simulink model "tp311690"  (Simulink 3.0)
settings: Solver=ode45  StartTime=0.0  StopTime=1  RelTol=1e-3

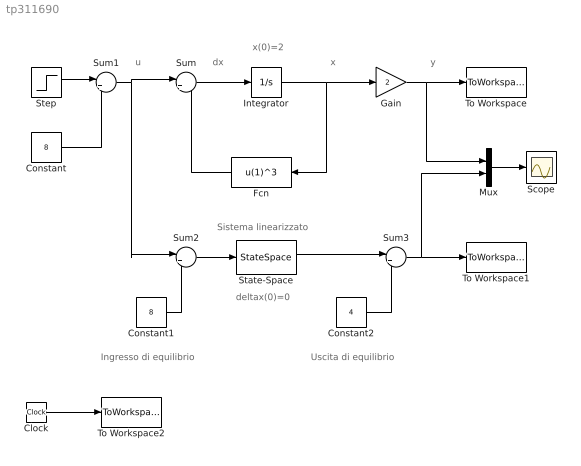
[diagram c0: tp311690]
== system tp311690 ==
  note: dx
  note: x
  note: y
  note: Sistema linearizzato
  note: x(0)=2
  note: deltax(0)=0
  note: Ingresso di equilibrio
  note: Uscita di equilibrio
  note: u
  Clock : Clock
  Constant : Constant  Value=8
  Constant1 : Constant  Value=8
  Constant2 : Constant  Value=4
  Fcn : Fcn  Orientation=left  Expr=u(1)^3
  Gain : Gain  Gain=2  SaturateOnIntegerOverflow=on
  Integrator : Integrator  ExternalReset=none  InitialConditionSource=internal  InitialCondition=2  LimitOutput=off  UpperSaturationLimit=inf  LowerSaturationLimit=-inf  ShowSaturationPort=off  ShowStatePort=off  AbsoluteTolerance=auto
  Mux : Mux  Inputs=2
  Scope : Scope
  State-Space : StateSpace  A=-12  B=1  C=2  D=0  X0=0
  Step : Step  Time=0.1  Before=0  After=1  SampleTime=0
  Sum : Sum  Inputs=|+-  SaturateOnIntegerOverflow=on
  Sum1 : Sum  Inputs=|++  SaturateOnIntegerOverflow=on
  Sum2 : Sum  Inputs=|+-  SaturateOnIntegerOverflow=on
  Sum3 : Sum  Inputs=|++  SaturateOnIntegerOverflow=on
  To Workspace : ToWorkspace  VariableName=y  SampleTime=-1  SaveFormat=Matrix
  To Workspace1 : ToWorkspace  VariableName=yl  SampleTime=-1  SaveFormat=Matrix
  To Workspace2 : ToWorkspace  VariableName=t  SampleTime=-1  SaveFormat=Matrix
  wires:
  Integrator/1 -> Gain/1, Fcn/1
  Sum/1 -> Integrator/1
  Gain/1 -> To Workspace/1, Mux/1
  Fcn/1 -> Sum/2
  Clock/1 -> To Workspace2/1
  Step/1 -> Sum1/1
  Sum1/1 -> Sum/1, Sum2/1
  Constant/1 -> Sum1/2
  Constant1/1 -> Sum2/2
  Sum2/1 -> State-Space/1
  State-Space/1 -> Sum3/1
  Constant2/1 -> Sum3/2
  Sum3/1 -> To Workspace1/1, Mux/2
  Mux/1 -> Scope/1
